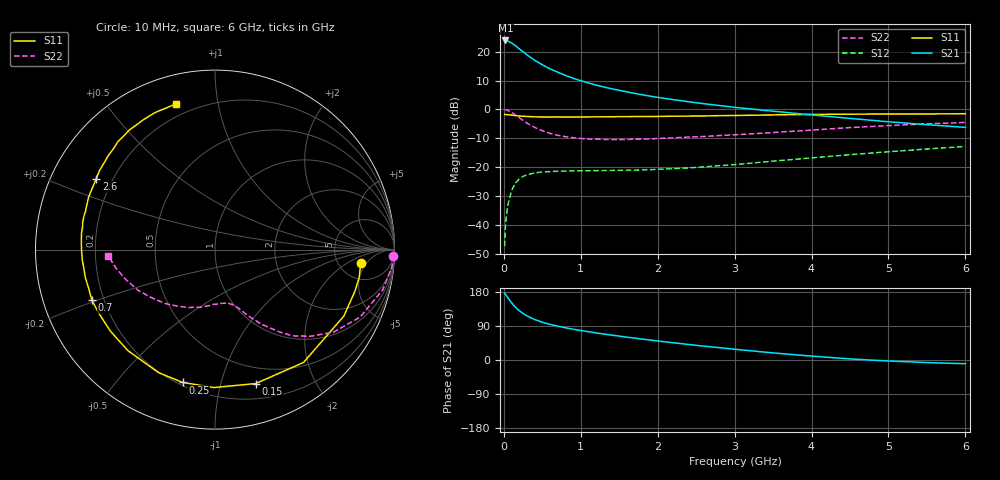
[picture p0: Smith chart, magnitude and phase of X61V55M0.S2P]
! SIEMENS Small Signal Semiconductors
! BFP193W
! Si NPN RF Bipolar Junction Transistor in SOT343
! VCE = 1.5 V  IC = 5 mA
! Common Emitter S-Parameters:  April 1994
# GHz  S  MA  R  50
!  f  S11  S21  S12  S22
! GHz  MAG  ANG  MAG  ANG  MAG  ANG  MAG  ANG
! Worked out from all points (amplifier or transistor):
!   40 points, 10 MHz to 6 GHz, reference 50 ohm
!   highest |S21| = 23.9 dB at 20 MHz (marker M1)
!   |S21| within 3 dB of that: start of sweep to 205.5 MHz
!   unconditionally stable (mu >= 1): 1.644 GHz to 4.762 GHz
!   at 200 MHz: K = 0.14, MSG = 22.5 dB, |S12| = -24.1 dB
!   at 1.5 GHz: K = 0.93, MSG = 13.8 dB, |S12| = -21.1 dB
!   at 6 GHz: K = 0.96, MSG = 3.3 dB, |S12| = -12.8 dB
!   S11 on the Smith chart (normalised r, x): 10 MHz: 8.11, -3.72; 150 MHz: 0.34, -1.29; 250 MHz: 0.22, -0.76; 700 MHz: 0.15, -0.19; 2.6 GHz: 0.14, +0.27; 6 GHz: 0.14, +0.76
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0.01  0.8155 -5.4  15.54 176.2  0.0043 87.1  0.994 -1.9
0.02  0.8182 -11.1  15.6 173.9  0.0089 82.4  0.9906 -5.6
0.03  0.8135 -16.6  15.53 171.0  0.0132 82.2  0.9786 -8.2
0.05  0.8078 -27.3  15.23 164.9  0.0216 76.0  0.961 -13.5
0.1  0.7991 -51.9  14.1 151.3  0.0392 64.1  0.8915 -25.0
0.15  0.7801 -73.1  12.69 139.4  0.0533 54.0  0.8043 -34.9
0.2  0.7685 -90.4  11.19 130.0  0.0626 46.5  0.7186 -42.2
0.25  0.7618 -103.7  9.932 122.6  0.0693 40.7  0.6457 -48.1
0.3  0.7542 -114.7  8.788 116.4  0.0736 36.1  0.5801 -52.1
0.4  0.7433 -130.9  7.108 106.9  0.0796 29.5  0.4887 -58.2
0.5  0.7389 -142.3  5.915 99.7  0.0826 25.9  0.4281 -62.2
0.6  0.7377 -150.9  5.035 94.0  0.084 23.2  0.3854 -65.4
0.7  0.7417 -157.6  4.403 89.3  0.0853 21.8  0.3564 -67.6
0.9  0.739 -167.7  3.469 81.3  0.0866 20.2  0.3231 -72.0
1.1  0.7414 -175.2  2.872 74.6  0.0872 20.0  0.3071 -76.1
1.6  0.7488 170.3  2.008 60.2  0.0887 22.9  0.3025 -86.7
2.2  0.7626 157.2  1.479 45.6  0.0942 29.1  0.321 -100.3
2.6  0.7704 149.2  1.255 36.6  0.1012 33.4  0.3395 -109.6
3.2  0.7922 138.6  1.023 24.6  0.117 38.0  0.3769 -123.1
4.5  0.826 119.1  0.699 2.8  0.1646 39.8  0.4845 -152.0
5.5  0.8342 109.5  0.544 -6.8  0.2065 36.2  0.5622 -169.6
6  0.8408 104.8  0.489 -9.8  0.2286 34.0  0.5947 -176.6
